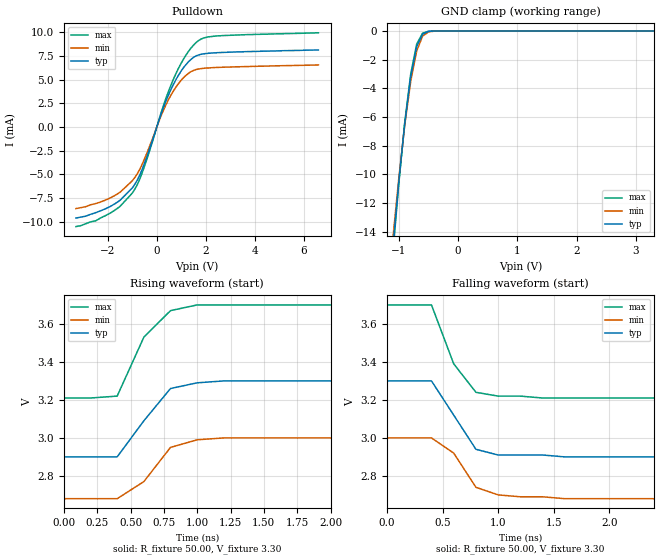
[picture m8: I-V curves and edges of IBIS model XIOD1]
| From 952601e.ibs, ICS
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|   Model XIOD1
[Model]   XIOD1
Model_type   I/O_open_drain
Polarity   Inverting
Enable   Active-High
Vinl =   0.80V
Vinh =   2.00V
C_comp   5.50pF   5.00pF   6.00pF
[Temperature Range]   25.00   70.00   1.00
[Voltage Range]   3.30V   3.00V   3.70V
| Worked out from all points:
|   slope of the pulldown table from 0 to 0.495 V, typ, clamps not added: 142 ohm
|   GND clamp passes 1 mA (typ) near -0.69 V on its own axis
|   rising waveform, R_fixture 50.00, V_fixture 3.30: 20-80 % time 269ps typ, 242ps min, 246ps max; typ from 2.9 V to 3.3 V
|   falling waveform, R_fixture 50.00, V_fixture 3.30: 20-80 % time 267ps typ, 236ps min, 246ps max; typ from 3.3 V to 2.9 V
[Pulldown]
| voltage   I(typ)   I(min)   I(max)
-3.3V     -9.6mA     -8.6mA     -10.5mA
-2.5V     -9.04mA    -8.08mA    -9.9mA
-1.9V     -8.38mA    -7.48mA    -9.08mA
-1.5V     -7.73mA    -6.88mA    -8.37mA
-1V       -6.43mA    -5.67mA    -6.97mA
-600mV    -4.49mA    -3.95mA    -4.86mA
200mV     1.55mA     1.34mA     1.7mA
700mV     4.6mA      3.89mA     5.17mA
1.2V      6.61mA     5.47mA     7.62mA
1.7V      7.6mA      6.12mA     9.11mA
2.5V      7.85mA     6.29mA     9.62mA
6.6V      8.13mA     6.55mA     9.94mA
[GND_clamp]
| voltage   I(typ)   I(min)   I(max)
-3.3V     -140mA     -130mA     -150mA
-1.1V     -15.07mA   -14.41mA   -15.48mA
-1V       -10.46mA   -10.24mA   -10.6mA
-900mV    -6.43mA    -6.54mA    -6.34mA
-800mV    -3.19mA    -3.51mA    -2.99mA
-700mV    -1.09mA    -1.4mA     -920uA
-600mV    -220uA     -360uA     -150uA
-500mV    -26.72uA   -59.35uA   -15.66uA
-400mV    -2.3uA     -7.36uA    -1.04uA
3.3V      140pA      520pA      120pA
[Ramp]
| variable   typ   min   max
dV/dt_r   0.24/0.17n   0.19/0.18n   0.29/0.19n
dV/dt_f   0.24/0.17n   0.19/0.19n   0.29/0.19n
R_load = 50.00
[Rising Waveform]
R_fixture = 50.00
V_fixture = 3.30
V_fixture_min = 3.00
V_fixture_max = 3.70
| time   V(typ)   V(min)   V(max)
0s        2.9V       2.68V      3.21V
200ps     2.9V       2.68V      3.21V
400ps     2.9V       2.68V      3.22V
600ps     3.09V      2.77V      3.53V
800ps     3.26V      2.95V      3.67V
1ns       3.29V      2.99V      3.7V
1.2ns     3.3V       3V         3.7V
10ns      3.3V       3V         3.7V
[Falling Waveform]
R_fixture = 50.00
V_fixture = 3.30
V_fixture_min = 3.00
V_fixture_max = 3.70
| time   V(typ)   V(min)   V(max)
0s        3.3V       3V         3.7V
400ps     3.3V       3V         3.7V
600ps     3.12V      2.92V      3.39V
800ps     2.94V      2.74V      3.24V
1ns       2.91V      2.7V       3.22V
1.2ns     2.91V      2.69V      3.22V
1.4ns     2.91V      2.69V      3.21V
1.6ns     2.9V       2.68V      3.21V
10ns      2.9V       2.68V      3.21V
